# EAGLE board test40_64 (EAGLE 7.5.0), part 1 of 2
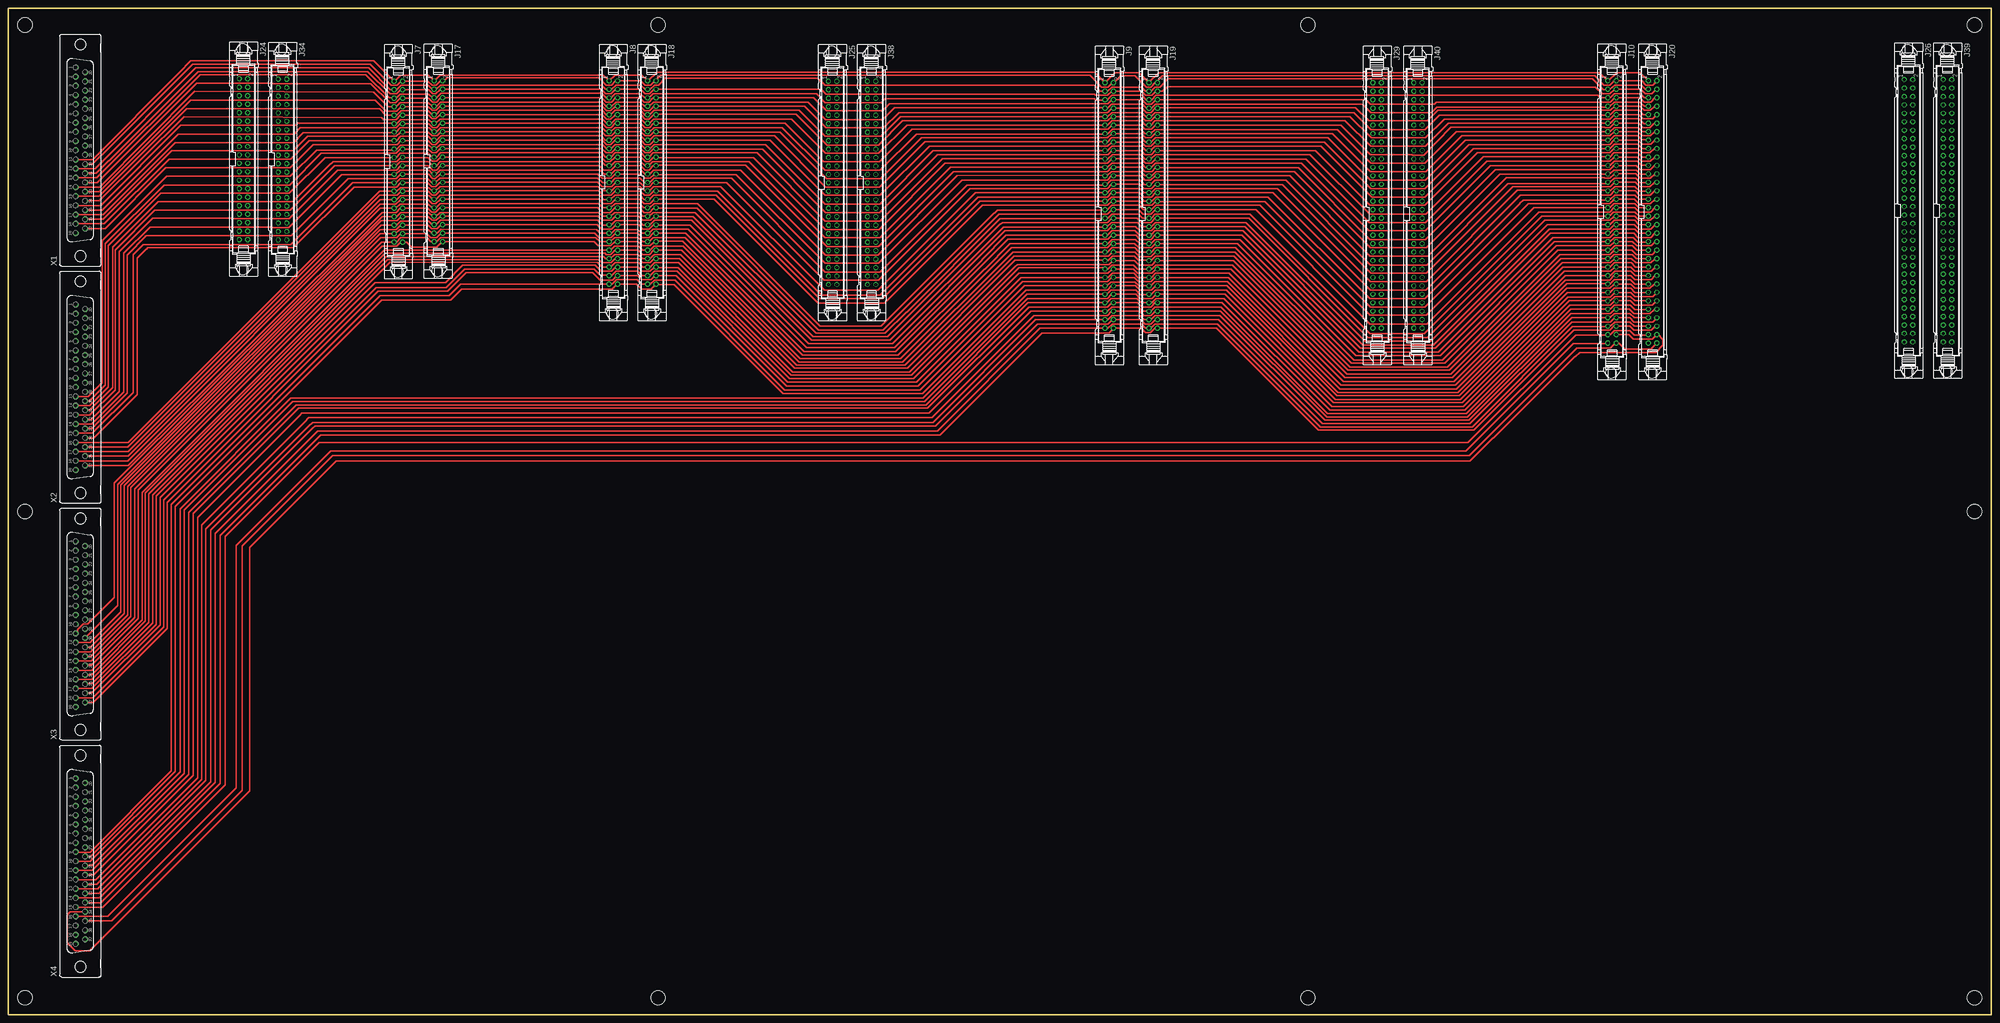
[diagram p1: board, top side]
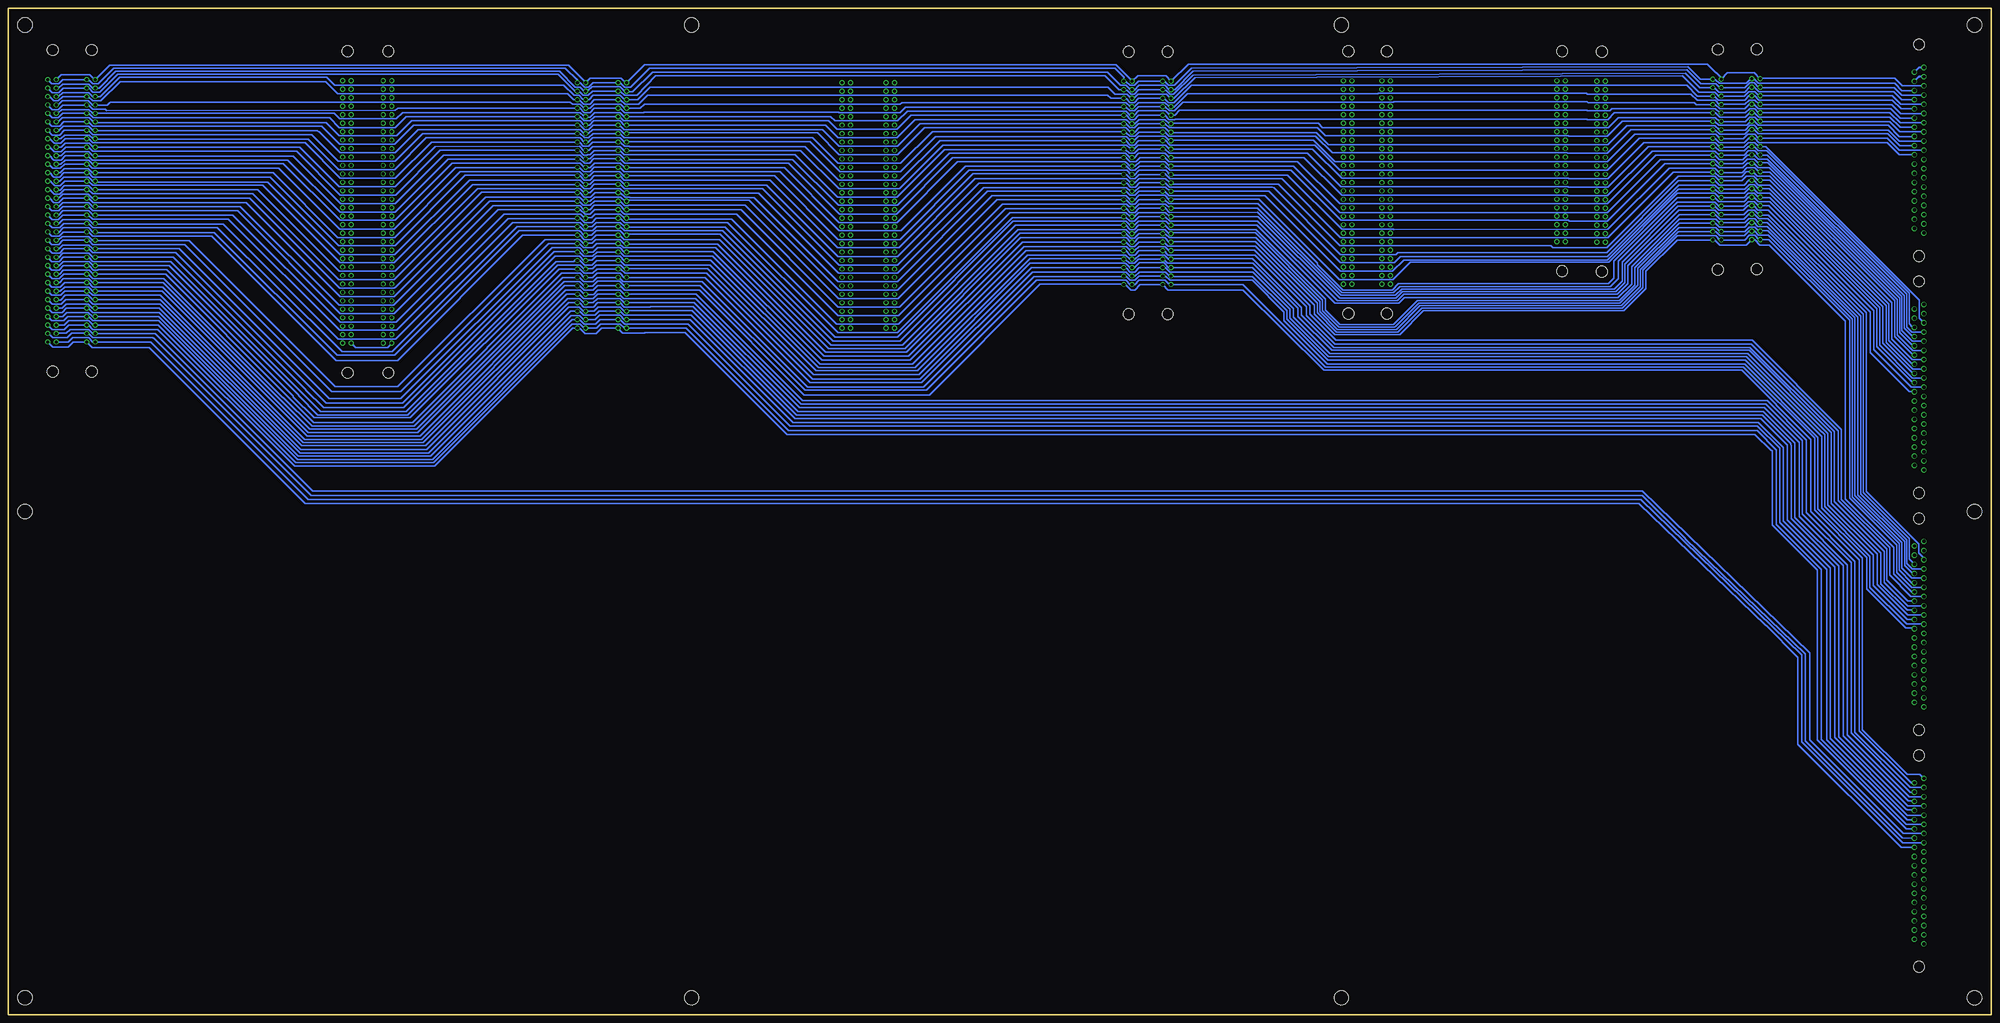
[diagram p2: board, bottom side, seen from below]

Size 595 x 302 mm. Coordinates in mm from the lower left corner, seen from the top.
Outline: 0,302 595,302 595,0 0,0 0,302
Copper layers (1*16): Top 0.035mm / dielectric 1.5mm / Bottom 0.035mm
Design rules "default": minimum track width 10mil, minimum drill 24mil, track to track 8mil, track to pad 8mil, pad to pad 8mil, via to via 8mil, smd to smd 8mil, copper to edge 40mil, drill to drill 8mil, minimum pad ring 10mil, minimum via ring 8mil, stop-mask expansion 4mil, vias tented up to drill 0mil, thermal gap 10mil
Holes 4.3 mm at 5,5 590,297 590,5 5,297 195,5 390,5 195,297 390,297 5,151 590,151

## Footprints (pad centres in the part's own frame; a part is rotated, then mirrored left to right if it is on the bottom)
40V = drill 0.914: 1 -24.13,-1.27 | drill 0.914 octagon: 2 -24.13,1.27; 3 -21.59,-1.27; 4 -21.59,1.27; 5 -19.05,-1.27; 6 -19.05,1.27; 7 -16.51,-1.27; 8 -16.51,1.27; 9 -13.97,-1.27; 10 -13.97,1.27; 11 -11.43,-1.27; 12 -11.43,1.27; 13 -8.89,-1.27; 14 -8.89,1.27; 15 -6.35,-1.27; 16 -6.35,1.27; 17 -3.81,-1.27; 18 -3.81,1.27; 19 -1.27,-1.27; 20 -1.27,1.27; 21 1.27,-1.27; 22 1.27,1.27; 23 3.81,-1.27; 24 3.81,1.27; 25 6.35,-1.27; 26 6.35,1.27; 27 8.89,-1.27; 28 8.89,1.27; 29 11.43,-1.27; 30 11.43,1.27; 31 13.97,-1.27; 32 13.97,1.27; 33 16.51,-1.27; 34 16.51,1.27; 35 19.05,-1.27; 36 19.05,1.27; 37 21.59,-1.27; 38 21.59,1.27; 39 24.13,-1.27; 40 24.13,1.27 | hole 3.302: 33.02,-0.254; -33.02,-0.254
50V = drill 0.914: 1 -30.48,-1.27 | drill 0.914 octagon: 2 -30.48,1.27; 3 -27.94,-1.27; 4 -27.94,1.27; 5 -25.4,-1.27; 6 -25.4,1.27; 7 -22.86,-1.27; 8 -22.86,1.27; 9 -20.32,-1.27; 10 -20.32,1.27; 11 -17.78,-1.27; 12 -17.78,1.27; 13 -15.24,-1.27; 14 -15.24,1.27; 15 -12.7,-1.27; 16 -12.7,1.27; 17 -10.16,-1.27; 18 -10.16,1.27; 19 -7.62,-1.27; 20 -7.62,1.27; 21 -5.08,-1.27; 22 -5.08,1.27; 23 -2.54,-1.27; 24 -2.54,1.27; 25 0,-1.27; 26 0,1.27; 27 2.54,-1.27; 28 2.54,1.27; 29 5.08,-1.27; 30 5.08,1.27; 31 7.62,-1.27; 32 7.62,1.27; 33 10.16,-1.27; 34 10.16,1.27; 35 12.7,-1.27; 36 12.7,1.27; 37 15.24,-1.27; 38 15.24,1.27; 39 17.78,-1.27; 40 17.78,1.27; 41 20.32,-1.27; 42 20.32,1.27; 43 22.86,-1.27; 44 22.86,1.27; 45 25.4,-1.27; 46 25.4,1.27; 47 27.94,-1.27; 48 27.94,1.27; 49 30.48,-1.27; 50 30.48,1.27 | hole 3.302: 39.37,-0.254; -39.37,-0.254
60V = drill 0.914: 1 -38.1,-1.27 | drill 0.914 octagon: 2 -38.1,1.27; 3 -35.56,-1.27; 4 -35.56,1.27; 5 -33.02,-1.27; 6 -33.02,1.27; 7 -30.48,-1.27; 8 -30.48,1.27; 9 -27.94,-1.27; 10 -27.94,1.27; 11 -25.4,-1.27; 12 -25.4,1.27; 13 -22.86,-1.27; 14 -22.86,1.27; 15 -20.32,-1.27; 16 -20.32,1.27; 17 -17.78,-1.27; 18 -17.78,1.27; 19 -15.24,-1.27; 20 -15.24,1.27; 21 -12.7,-1.27; 22 -12.7,1.27; 23 -10.16,-1.27; 24 -10.16,1.27; 25 -7.62,-1.27; 26 -7.62,1.27; 27 -5.08,-1.27; 28 -5.08,1.27; 29 -2.54,-1.27; 30 -2.54,1.27; 31 0,-1.27; 32 0,1.27; 33 2.54,-1.27; 34 2.54,1.27; 35 5.08,-1.27; 36 5.08,1.27; 37 7.62,-1.27; 38 7.62,1.27; 39 10.16,-1.27; 40 10.16,1.27; 41 12.7,-1.27; 42 12.7,1.27; 43 15.24,-1.27; 44 15.24,1.27; 45 17.78,-1.27; 46 17.78,1.27; 47 20.32,-1.27; 48 20.32,1.27; 49 22.86,-1.27; 50 22.86,1.27; 51 25.4,-1.27; 52 25.4,1.27; 53 27.94,-1.27; 54 27.94,1.27; 55 30.48,-1.27; 56 30.48,1.27; 57 33.02,-1.27; 58 33.02,1.27; 59 35.56,-1.27; 60 35.56,1.27
64V = drill 0.914: 1 -39.37,-1.27 | drill 0.914 octagon: 2 -39.37,1.27; 3 -36.83,-1.27; 4 -36.83,1.27; 5 -34.29,-1.27; 6 -34.29,1.27; 7 -31.75,-1.27; 8 -31.75,1.27; 9 -29.21,-1.27; 10 -29.21,1.27; 11 -26.67,-1.27; 12 -26.67,1.27; 13 -24.13,-1.27; 14 -24.13,1.27; 15 -21.59,-1.27; 16 -21.59,1.27; 17 -19.05,-1.27; 18 -19.05,1.27; 19 -16.51,-1.27; 20 -16.51,1.27; 21 -13.97,-1.27; 22 -13.97,1.27; 23 -11.43,-1.27; 24 -11.43,1.27; 25 -8.89,-1.27; 26 -8.89,1.27; 27 -6.35,-1.27; 28 -6.35,1.27; 29 -3.81,-1.27; 30 -3.81,1.27; 31 -1.27,-1.27; 32 -1.27,1.27; 33 1.27,-1.27; 34 1.27,1.27; 35 3.81,-1.27; 36 3.81,1.27; 37 6.35,-1.27; 38 6.35,1.27; 39 8.89,-1.27; 40 8.89,1.27; 41 11.43,-1.27; 42 11.43,1.27; 43 13.97,-1.27; 44 13.97,1.27; 45 16.51,-1.27; 46 16.51,1.27; 47 19.05,-1.27; 48 19.05,1.27; 49 21.59,-1.27; 50 21.59,1.27; 51 24.13,-1.27; 52 24.13,1.27; 53 26.67,-1.27; 54 26.67,1.27; 55 29.21,-1.27; 56 29.21,1.27; 57 31.75,-1.27; 58 31.75,1.27; 59 34.29,-1.27; 60 34.29,1.27; 61 36.83,-1.27; 62 36.83,1.27; 63 39.37,-1.27; 64 39.37,1.27 | hole 3.302: 48.26,-0.254; -48.26,-0.254
F37V = drill 1.016 octagon: 1 24.841,1.422; 2 22.073,1.422; 3 19.329,1.422; 4 16.561,1.422; 5 13.792,1.422; 6 11.049,1.422; 7 8.28,1.422; 8 5.512,1.422; 9 2.769,1.422; 10 0,1.422; 11 -2.769,1.422; 12 -5.512,1.422; 13 -8.28,1.422; 14 -11.049,1.422; 15 -13.818,1.422; 16 -16.561,1.422; 17 -19.329,1.422; 18 -22.098,1.422; 19 -24.841,1.422; 20 23.47,-1.422; 21 20.701,-1.422; 22 17.932,-1.422; 23 15.189,-1.422; 24 12.421,-1.422; 25 9.652,-1.422; 26 6.909,-1.422; 27 4.14,-1.422; 28 1.372,-1.422; 29 -1.372,-1.422; 30 -4.14,-1.422; 31 -6.909,-1.422; 32 -9.677,-1.422; 33 -12.421,-1.422; 34 -15.189,-1.422; 35 -17.958,-1.422; 36 -20.701,-1.422; 37 -23.47,-1.422 | hole 3.302: 31.75,0; -31.75,0

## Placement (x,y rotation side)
J7  [40V]  117.06,255.98 270 top
J8  [50V]  181.56,249.74 270 top
J9  60V  [60V]  330.38,241.56 270 top
J10  [64V]  481.2,240.88 270 top
J17  [40V]  129.03,256.11 270 top
J18  [50V]  193.13,249.74 270 top
J19  60V  [60V]  343.58,241.56 270 top
J20  [64V]  493.4,240.88 270 top
J24  [40V]  70.59,256.73 270 top
J25  [50V]  247.33,249.61 270 top
J26  [64V]  570.23,241.25 270 top
J29  60V  [60V]  410.78,241.56 270 top
J34  [40V]  82.31,256.63 270 top
J38  [50V]  259.03,249.61 270 top
J39  [64V]  581.93,241.25 270 top
J40  60V  [60V]  422.98,241.56 270 top
X1  [F37V]  21.63,259.4 90 top
X2  [F37V]  21.63,188.28 90 top
X3  [F37V]  21.63,117.16 90 top
X4  [F37V]  21.63,46.04 90 top

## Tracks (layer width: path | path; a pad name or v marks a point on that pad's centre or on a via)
1
  Bottom 0.406: X1.3 26.73,278.73 29,281 69.18,281 J24.1 69.36,280.86 71.12,282.62 79.17,282.62 J34.1 81.03,281.16 82.5,282.62 82.62,282.62 85.25,285.25 240.9,285.25 J25.1 246.06,280.19 247.62,281.75 256.1,281.75 J38.1 257.76,280.26 262.62,285.12 | J29.1 409.79,279.67 411.12,281 420.38,281 J40.1
  Bottom 0.506: J40.1 421.71,279.83 426.88,285 564.58,285 J26.1 569.12,280.62 570.62,282.12 579.15,282.12 J39.1
  Bottom 0.51: 262.62,285.12 404.05,285.12 J29.1
2
  Bottom 0.406: X1.22 26.83,277.33 29,279.5 69.88,279.5 71.23,280.86 J24.2 72.14,280.86 73.5,279.5 81.62,279.5 82.75,280.62 83.44,280.62 J34.2 87.27,280.76 91,284.49 240,284 245.12,278.88 246.88,278.88 248,280 248.51,280 J25.2 255.91,280.09 257.12,278.88 258.5,278.88 259.62,280 260.21,280 J38.2 | J29.2 419.58,279.67 420.88,278.38 422.12,278.38 423.38,279.62 424.21,279.62 J40.2
  Bottom 0.506: J40.2 424.25,280.38 427.88,284 563.38,284 568,279.38 569.75,279.38 570.62,280.25 571.13,280.25 J26.2 578.63,280.62 579.88,279.38 581.96,279.38 J39.2
  Bottom 0.51: J38.2 260.3,281.3 263,284 402.62,284 408.25,278.38 410.12,278.38 411.38,279.62 412.01,279.62 J29.2
3
  Bottom 0.406: X1.4 26.84,275.96 29.12,278.25 69.25,278.25 J24.3 69.82,278.32 71.12,279.62 72.38,279.62 73.88,278.12 80.94,278.12 J34.3 81.47,278.22 82.62,279.38 87.14,279.38 91.38,283.61 239.5,283.12 245,277.62 245.99,277.62 J25.3 246.68,277.55 248,278.88 255.75,278.88 257.12,277.5 257.71,277.5 J38.3 | J29.3 410.12,277.12 411.5,278.5 419.88,278.5 421.12,277.25 421.58,277.25 J40.3 | J26.3 569.71,278.08 570.88,279.25 578.75,279.25 580,278 580.58,278 J39.3
  Bottom 0.506: J26.3 567.79,278.08 562.75,283.12 429.62,283.12 424.88,278.38 423.5,278.38 422.25,277.12 J40.3
  Bottom 0.51: J38.3 258.3,277.55 259.62,278.88 261.25,278.88 265.25,282.88 401.75,282.88 407.62,277 409.38,277 J29.3
4
  Bottom 0.406: X1.23 26.84,274.59 29.25,277 69.75,277 71.12,278.38 71.81,278.38 J24.4 | J24.4 71.86,278.26 | J24.4 72.56,278.32 74,276.88 81.75,276.88 82.88,278 83.36,278 J34.4 87.48,278.22 91.75,282.49 239.5,282 245.38,276.25 246.38,276.25 247.62,277.38 248.43,277.38 J25.4 255.82,277.55 257.12,276.25 258.12,276.25 259.38,277.5 260.25,277.5 J38.4 | J29.4 419.75,277.12 421,275.88 422.5,275.88 423.62,277 424.12,277 J40.4 | J26.4 578.54,278.08 579.88,276.75 581.87,276.75 J39.4
  Bottom 0.506: J40.4 424.88,277.12 430,282.25 562.25,282.25 567.62,276.88 569.62,276.88 570.75,278 571.42,278 J26.4
  Bottom 0.51: J38.4 261.8,277.55 266,281.75 400.75,281.75 406.38,276 406.5,275.88 410.12,275.88 411.25,277 411.93,277 J29.4
5
  Bottom 0.406: X1.5 27.07,273.19 29.62,275.75 69.29,275.75 J24.5 69.78,275.78 71,277 72.75,277 74.12,275.62 80.98,275.62 J34.5 81.68,275.68 82.88,276.88 87.76,276.88 92.62,281.74 239,281.25 245.25,275 J25.5 246.26,275.01 247.5,276.25 256,276.25 257.12,275.12 257.64,275.12 J38.5 | J29.5 410.08,274.58 411.38,275.88 419.5,275.88 420.75,274.62 421.67,274.62 J40.5 | J26.5 569.66,275.54 570.88,276.75 578.75,276.75 579.88,275.62 580.58,275.62 J39.5
  Bottom 0.506: J26.5 567.46,275.54 561.62,281.38 499.5,281.38 497.12,279 428.38,279 425.25,275.88 423.75,275.88 422.62,274.75 421.88,274.75 J40.5
  Bottom 0.51: J38.5 258.13,275.01 259.38,276.25 262.88,276.25 265,278.38 402.38,278.38 406.12,274.62 409.47,274.62 J29.5
6
  Bottom 0.406: X1.24 26.95,271.82 29.62,274.5 69.75,274.5 71,275.75 71.83,275.75 J24.6 72.72,275.78 74,274.5 81.88,274.5 82.88,275.5 83.39,275.5 J34.6 88.18,275.68 91.38,278.88 121.25,278.88 121.38,279 240,279 245.25,273.75 246.88,273.75 247.88,274.75 248.34,274.75 J25.6 255.87,275.01 257.12,273.75 258.38,273.75 259.5,274.88 260.17,274.88 J38.6 | J29.6 419.17,274.58 420.5,273.25 422.38,273.25 423.62,274.5 424.17,274.5 J40.6 | J26.6 578.71,275.54 580,274.25 581.38,274.25 582.62,275.5 583.16,275.5 J39.6
  Bottom 0.506: J40.6 425.33,274.58 427.12,276.38 496.12,276.38 499.75,280 561.5,280 567.25,274.25 569.75,274.25 571,275.5 571.46,275.5 J26.6
  Bottom 0.51: J38.6 264.13,275.01 265.12,276 327.88,276 328,275.88 403.25,275.88 405.88,273.25 410,273.25 411.25,274.5 411.96,274.5 J29.6
7
  Bottom 0.406: X1.6 27.2,270.45 29.88,273.12 69.2,273.12 J24.7 69.61,273.24 70.88,274.5 72.62,274.5 73.88,273.25 80.92,273.25 J34.7 81.52,273.14 82.75,274.38 88.25,274.38 90.12,276.25 121.25,276.25 121.5,276.5 183.88,276.5 184,276.38 241.25,276.38 245.25,272.38 245.97,272.38 J25.7 246.59,272.47 247.88,273.75 255.88,273.75 257.25,272.38 257.67,272.38 J38.7 | J29.7 410.05,272.05 411.25,273.25 419.25,273.25 420.5,272 421.67,272 J40.7 | J26.7 569.75,273 571,274.25 578.88,274.25 579.88,273.25 580.41,273.25 J39.7
  Bottom 0.506: J26.7 565.38,273 564.62,273.75 564.5,273.75 564.38,273.88 426.38,273.88 425.75,273.25 423.5,273.25 422.38,272.12 421.79,272.12 J40.7
  Bottom 0.51: J38.7 258.35,272.47 259.62,273.75 326.88,273.75 327.38,273.25 404.12,273.25 405.38,272 409.46,272 J29.7
8
  Bottom 0.406: X1.25 27.3,269.05 30.12,271.88 69.87,271.88 71.23,273.24 J24.8 72.64,273.24 74,271.88 81.5,271.88 82.75,273.12 83.56,273.12 J34.8 88.52,273.14 89.12,273.75 121,273.75 121.25,274 179.25,274 179.38,273.88 242.5,273.88 245.12,271.25 246.62,271.25 247.88,272.5 248.57,272.5 J25.8 255.91,272.47 257.12,271.25 258.5,271.25 259.62,272.38 260.2,272.38 J38.8 | J29.8 419.2,272.05 420.5,270.75 422.25,270.75 423.62,272.12 424.17,272.12 J40.8 | J26.8 578.62,273 580,271.62 581.83,271.62 J39.8
  Bottom 0.506: J26.8 571.38,272.88 570.88,272.88 569.75,271.75 566,271.75 565.5,271.25 478.88,271.38 478.08,272.05 J40.8
  Bottom 0.51: J29.8 411.42,272.05 410.12,270.75 404.38,270.75 404.25,270.88 345.88,270.88 345.75,270.75 327.38,270.75 325.75,272.38 260.39,272.38 J38.8
9
  Bottom 0.406: X1.7 27.3,267.68 30.38,270.75 69.27,270.75 J24.9 69.83,270.7 71,271.88 72.5,271.88 73.75,270.62 81.01,270.62 J34.9 81.47,270.6 82.75,271.88 113.88,271.88 114.5,271.25 121.12,271.25 121.38,271.38 179.5,271.5 179.62,271.38 243.62,271.38 245,270 245.99,270 J25.9 246.43,269.93 247.75,271.25 255.88,271.25 257.12,270 257.69,270 J38.9 | J29.9 410.25,269.5 411.5,270.75 419.12,270.75 420.5,269.38 421.58,269.38 J40.9 | J26.9 569.71,270.46 570.88,271.62 579,271.62 580,270.62 580.5,270.62 J39.9
  Bottom 0.506: J40.9 421.95,269.75 422.38,269.75 423.38,270.75 476.75,270.75 478.62,268.88 495.62,268.88 | 495.75,268.88 495.62,268.88 | J26.9 497.21,270.46 495.62,268.88
  Bottom 0.51: J38.9 258.43,269.93 259.62,271.12 325.25,271.12 328.12,268.25 347,268.25 348.25,269.5 J29.9
10
  Bottom 0.406: X1.26 27.31,266.31 30.38,269.38 69.75,269.38 71.12,270.75 71.81,270.75 J24.10 72.42,270.7 73.75,269.38 81.5,269.38 82.75,270.62 83.55,270.62 J34.10 113.03,270.6 115,268.62 121.25,268.62 121.38,268.75 244.88,268.75 245,268.62 246.75,268.62 248,269.88 248.54,269.88 J25.10 255.82,269.93 257.12,268.62 258.25,268.62 259.5,269.88 260.25,269.88 J38.10 | J29.10 419.12,269.5 420.38,268.25 422.25,268.25 423.5,269.5 J40.10 | J26.10 578.66,270.46 580,269.12 581.87,269.12 J39.10
  Bottom 0.506: J40.10 475.62,269.5 478.88,266.25 495.75,266.25 498.62,269.12 569.5,269.12 570.88,270.5 571.46,270.5 J26.10
  Bottom 0.51: J29.10 411.63,269.5 410.38,268.25 348.88,268.25 346.38,265.75 328.38,265.75 324.12,270 260.37,270 J38.10
11
  Bottom 0.406: X1.8 27.41,264.91 30.5,268 69.16,268 J24.11 69.78,268.16 71,269.38 72.38,269.38 73.75,268 80.97,268 J34.11 81.56,268.06 82.75,269.25 111.88,269.25 114.88,266.25 200.62,266.25 201.88,267.5 245.95,267.5 J25.11 246.64,267.39 247.88,268.62 255.75,268.62 257.12,267.25 257.62,267.25 J38.11 | J29.11 410.21,266.96 411.5,268.25 419.38,268.25 420.62,267 421.68,267 J40.11 | J26.11 569.54,267.92 570.75,269.12 578.88,269.12 580.12,267.88 580.62,267.88 J39.11
  Bottom 0.506: J40.11 422.21,266.96 423.5,268.25 474,268.25 478.5,263.75 495.75,263.75 499.62,267.62 568.66,267.62 J26.11
  Bottom 0.51: J38.11 258.26,267.39 259.38,268.5 259.5,268.5 259.62,268.62 322.88,268.62 328.38,263.12 346,263.12 349.75,266.88 409.42,266.88 J29.11
12
  Bottom 0.406: X1.27 27.54,263.54 30.88,266.88 69.88,266.88 71.12,268.12 71.83,268.12 J24.12 72.09,268.16 73.38,266.88 81.75,266.88 82.88,268 83.52,268 J34.12 110.69,268.06 115.12,263.62 126.75,263.62 126.88,263.75 199.75,263.75 202.12,266.12 246.62,266.12 247.88,267.38 248.59,267.38 J25.12 255.86,267.39 257.12,266.12 258.38,266.12 259.62,267.38 260.29,267.38 J38.12 | J29.12 419.54,266.96 420.88,265.62 422.12,265.62 423.38,266.88 424.16,266.88 J40.12 | J26.12 578.33,267.92 579.62,266.62 581.9,266.62 J39.12
  Bottom 0.506: J40.12 473.41,266.96 479.12,261.25 495.62,261.25 501,266.62 569.62,266.62 570.88,267.88 571.46,267.88 J26.12
  Bottom 0.51: J29.12 411.59,266.96 410.25,265.62 350.75,265.62 345.75,260.62 328.25,260.62 321.5,267.38 260.31,267.38 J38.12
13
  Bottom 0.406: X1.9 27.54,262.17 30.88,265.5 69.2,265.5 J24.13 69.87,265.62 71.12,266.88 72.38,266.88 73.75,265.5 81.02,265.5 J34.13 81.64,265.52 82.88,266.75 109.38,266.75 115,261.12 198.88,261.12 202.5,264.75 245.96,264.75 J25.13 246.6,264.85 247.88,266.12 255.75,266.12 257,264.88 257.74,264.88 J38.13 | J29.13 410.3,264.43 411.5,265.62 419.75,265.62 420.88,264.5 421.63,264.5 J40.13 | J26.13 569.63,265.38 570.88,266.62 578.5,266.62 579.88,265.25 580.53,265.25 J39.13
  Bottom 0.506: J40.13 422.18,264.43 423.38,265.62 472,265.62 479,258.62 495.38,258.62 501.75,265 502,265 502.25,265.25 568.83,265.25 J26.13
  Bottom 0.51: J38.13 258.35,264.85 259.62,266.12 320.12,266.12 328.25,258.12 345.75,258.12 352.25,264.62 409.31,264.62 J29.13
14
  Bottom 0.406: X1.28 27.4,260.77 31,264.38 69.88,264.38 71.12,265.62 J24.14 72.63,265.62 74,264.25 81.5,264.25 82.75,265.5 83.56,265.5 J34.14 108.11,265.52 115.12,258.5 127.12,258.5 127.25,258.62 197.75,258.62 202.75,263.62 246.75,263.62 248,264.88 248.57,264.88 J25.14 255.78,264.85 257,263.62 258.5,263.62 259.62,264.75 260.2,264.75 J38.14 | J29.14 419.57,264.43 420.88,263.12 422.12,263.12 423.38,264.38 424.2,264.38 J40.14 | J26.14 578.25,265.38 579.62,264 581.82,264 J39.14
  Bottom 0.506: J40.14 470.7,264.43 479,256.12 496,256.12 504,264.12 569.62,264.12 570.88,265.25 571.37,265.25 J26.14
  Bottom 0.51: J29.14 411.43,264.43 410.25,263.25 353.75,263.25 346,255.5 327.25,255.5 317.75,265 260.45,265 J38.14
15
  Bottom 0.406: X1.10 27.52,259.4 31.12,263 69.24,263 J24.15 69.83,263.08 71,264.25 73,264.25 74.38,262.88 80.93,262.88 J34.15 81.36,262.98 82.62,264.25 107,264.25 115.25,256 196.88,256 203.38,262.5 245.87,262.5 J25.15 246.56,262.31 247.88,263.62 255.88,263.62 257.25,262.25 257.7,262.25 J38.15 | J29.15 410.13,261.88 411.38,263.12 419.75,263.12 421,261.88 J40.15 | J26.15 569.59,262.84 570.75,264 578.12,264 579.25,262.88 580.62,262.88 J39.15
  Bottom 0.506: J40.15 422.26,261.88 423.5,263.12 469.62,263.12 479.12,253.62 495.88,253.62 505,262.75 568.87,262.75 J26.15
  Bottom 0.51: J38.15 258.31,262.31 259.5,263.5 316.75,263.5 327.25,253 345.5,253 354.5,262 409.39,262 J29.15
16
  Bottom 0.406: X1.29 27.53,258.03 31.25,261.75 69.75,261.75 71,263 71.78,263 J24.16 72.8,263.08 74.12,261.75 81.62,261.75 82.75,262.88 83.47,262.88 J34.16 105.64,262.98 115.25,253.38 126.75,253.38 126.88,253.5 195.5,253.5 203,261 246.38,261 247.75,262.38 248.53,262.38 J25.16 255.81,262.31 257.12,261 258.38,261 259.62,262.25 260.24,262.25 J38.16 | J29.16 419.62,261.88 420.88,260.62 422.5,260.62 423.5,261.62 | 423.75,261.88 J40.16 | J26.16 577.91,262.84 579.25,261.5 581.25,261.5 582.62,262.88 583.16,262.88 J39.16
  Bottom 0.506: J26.16 570.84,262.84 569.62,261.62 506,261.62 495.38,251 478.88,251 468,261.88 423.75,261.88 423.5,261.62
  Bottom 0.51: J38.16 315.44,262.31 327.38,250.38 345.88,250.38 356,260.5 408.62,260.5 408.75,260.62 410.12,260.62 411.25,261.75 411.92,261.75 J29.16
17
  Bottom 0.406: X2.3 20.23,207.61 21.62,209 21.62,214.5 67.62,260.5 69.28,260.5 J24.17 69.79,260.54 71,261.75 72.88,261.75 74.25,260.38 80.97,260.38 J34.17 81.56,260.44 82.75,261.62 104.25,261.62 115,250.88 126.75,250.88 126.88,251 194.88,251 203.62,259.75 246.04,259.75 J25.17 246.52,259.77 247.75,261 256,261 257.12,259.88 257.65,259.88 J38.17 | J29.17 410.22,259.35 411.38,260.5 419.62,260.5 420.75,259.38 421.68,259.38 J40.17 | J26.17 569.55,260.3 570.75,261.5 578,261.5 579.12,260.38 580.59,260.38 J39.17
  Bottom 0.506: J40.17 422.35,259.35 423.62,260.62 466.88,260.5 478.88,248.5 495.75,248.5 507.62,260.38 568.88,260.38 J26.17
  Bottom 0.51: J29.17 357.22,259.35 345.75,247.88 327.62,247.88 314.5,261 259.5,261 258.5,260 257.99,260 J38.17
18
  Bottom 0.406: X2.22 23.21,206.38 23.62,206.38 24.62,207.38 24.62,216.5 67.38,259.25 69.88,259.25 71,260.38 71.69,260.38 J24.18 72.83,260.54 74.12,259.25 81.62,259.25 82.75,260.38 83.51,260.38 J34.18 102.94,260.44 115,248.38 126.88,248.38 127,248.5 195.12,248.5 205.12,258.5 246.62,258.5 247.88,259.75 248.58,259.75 J25.18 255.85,259.77 257.12,258.5 258.62,258.5 259.75,259.62 260.15,259.62 J38.18 | J29.18 419.28,259.35 420.5,258.12 421.25,258.12 421.38,258 422.38,258 423.62,259.25 424.15,259.25 J40.18 | J26.18 577.83,260.3 579.12,259 581.25,259 582.62,260.38 583.12,260.38 J39.18
  Bottom 0.506: J26.18 570.92,260.3 569.75,259.12 508.5,259.12 495.38,246 478.75,246 465.38,259.38 424.28,259.38 J40.18
  Bottom 0.51: J29.18 411.47,259.35 410.25,258.12 358.88,258.12 346.12,245.38 328.38,245.38 314.12,259.62 260.44,259.62 J38.18
19
  Bottom 0.406: X2.4 23.84,204.84 25.38,206.38 25.38,216.25 67.12,258 J24.19 69.75,258 71,259.25 72.88,259.25 74.12,258 80.94,258 J34.19 81.65,257.9 82.88,259.12 101.75,259.12 115.12,245.75 126.88,245.75 127,245.88 194.88,245.88 206.25,257.25 246.04,257.25 J25.19 246.6,257.23 247.88,258.5 255.88,258.5 257.12,257.25 257.74,257.25 J38.19 | J29.19 410.18,256.81 411.5,258.12 419.25,258.12 420.5,256.88 421.64,256.88 J40.19 | J26.19 569.63,257.76 570.88,259 577.88,259 579.12,257.75 J39.19
  Bottom 0.506: J40.19 422.31,256.81 423.5,258 464.38,258 479,243.38 495.25,243.38 509.5,257.62 568.83,257.62 J26.19
  Bottom 0.51: J38.19 258.48,257.23 259.75,258.5 312.62,258.5 328.25,242.88 345.88,242.88 359.62,256.62 409.33,256.62 J29.19
20
  Bottom 0.406: X2.23 23.59,203.47 26.12,206 26.12,215.75 67.12,256.75 69.88,256.75 71.12,258 J24.20 73.12,258 74.5,256.62 81.62,256.62 82.75,257.75 83.42,257.75 J34.20 100.6,257.9 115.12,243.38 195.5,243.38 208.12,256 246.75,256 248,257.25 248.58,257.25 J25.20 255.4,257.23 256.62,256 258.5,256 259.62,257.12 260.19,257.12 J38.20 | J29.20 419.32,256.81 420.62,255.5 422.12,255.5 423.38,256.75 423.75,256.75 424.19,256.75 J40.20 | J26.20 577.87,257.76 579.12,256.5 581.38,256.5 582.62,257.75 J39.20
  Bottom 0.506: J26.20 571.13,257.76 569.88,256.5 511.12,256.5 495.5,240.88 478.88,240.88 463,256.75 423.75,256.75
  Bottom 0.51: J29.20 411.43,256.81 410.12,255.5 360.88,255.5 345.62,240.25 328.5,240.25 311.62,257.12 260.4,257.12 J38.20
21
  Bottom 0.406: X2.5 23.7,202.07 26.88,205.25 26.88,215.5 67,255.62 69.16,255.62 J24.21 69.83,255.46 71.12,256.75 73.12,256.75 74.5,255.38 81.02,255.38 J34.21 81.73,255.36 83,256.62 99.25,256.62 115.25,240.62 126.88,240.62 127,240.75 195.5,240.75 209.38,254.62 246,254.62 J25.21 246.56,254.69 247.88,256 255.5,256 256.88,254.62 257.69,254.62 J38.21 | J29.21 410.14,254.26 411.38,255.5 419.12,255.5 420.5,254.12 421.57,254.12 J40.21 | 569.5,255.12 570.88,256.5 578,256.5 579.25,255.25 580.63,255.25 J39.21
  Bottom 0.506: J40.21 422.26,254.26 423.5,255.5 461.88,255.5 479,238.38 495.5,238.38 512.5,255.38 569.25,255.38 569.5,255.12 569.05,255.12 J26.21
  Bottom 0.51: J38.21 258.44,254.69 259.62,255.88 259.75,255.88 259.88,256 310.12,256 328.38,237.75 345.75,237.75 362.12,254.12 409.37,254.12 J29.21
22
  Bottom 0.406: X2.24 23.45,200.7 27.5,204.75 27.5,215 66.62,254.12 69.88,254.12 71.12,255.38 71.78,255.38 J24.22 73.17,255.46 74.5,254.12 81.62,254.12 82.75,255.25 83.47,255.25 J34.22 97.89,255.36 115.12,238.12 126.62,238.12 126.88,238.38 195.12,238.38 210.12,253.38 246.5,253.38 247.75,254.62 248.53,254.62 J25.22 255.56,254.69 256.88,253.38 258.25,253.38 259.5,254.62 260.24,254.62 J38.22 | J29.22 419.24,254.26 420.5,253 422.38,253 423.62,254.25 424.24,254.25 J40.22 | J39.22 582.85,255.22 581.62,254 579.38,254 578.12,255.25 571.53,255.25 J26.22
  Bottom 0.506: J26.22 571.1,255.22 569.88,254 513.88,254 495.62,235.75 479.25,235.75 460.75,254.25 424.26,254.25 J40.22
  Bottom 0.51: J29.22 411.51,254.26 410.25,253 363.5,253 345.75,235.25 327.12,235.25 307.75,254.62 260.37,254.62 J38.22
23
  Bottom 0.406: X2.6 23.58,199.33 28.25,204 28.25,214.62 66.5,252.88 69.28,252.88 J24.23 69.8,252.92 71,254.12 73.38,254.12 74.75,252.75 80.97,252.75 J34.23 81.69,252.82 82.88,254 96.62,254 115,235.75 179.25,235.62 179.38,235.75 194.88,235.75 211.12,252 245.91,252 J25.23 246.4,252.15 247.62,253.38 255.75,253.38 257.12,252 257.61,252 J38.23 | J29.23 410.35,251.72 411.62,253 419.38,253 420.62,251.75 421.69,251.75 J40.23 | J26.23 569.8,252.68 571,253.88 578.25,253.88 579.5,252.62 580.61,252.62 J39.23
  Bottom 0.506: J40.23 422.35,251.72 423.62,253 459.38,253 479.12,233.25 496.12,233.25 515.5,252.62 568.9,252.62 J26.23
  Bottom 0.51: J38.23 258.15,252.15 259.38,253.38 306.75,253.38 327.5,232.62 346,232.62 365.12,251.75 409.49,251.75 J29.23
24
  Bottom 0.406: X2.25 23.43,197.93 29,203.5 29,214.25 66.38,251.62 70.12,251.62 71.25,252.75 71.69,252.75 J24.24 73.45,252.92 74.88,251.5 81.62,251.5 82.88,252.75 83.5,252.75 J34.24 95.31,252.82 115,233.12 126.62,233.12 126.75,233.25 195.25,233.25 212.88,250.88 246.5,250.88 248,252.38 248.38,252.38 J25.24 255.72,252.15 257,250.88 258.25,250.88 259.5,252.12 260.27,252.12 J38.24 | J29.24 419.27,251.72 420.5,250.5 422.25,250.5 423.5,251.75 424.23,251.75 J40.24 | J26.24 578.32,252.68 579.62,251.38 581.38,251.38 582.62,252.62 583.14,252.62 J39.24
  Bottom 0.506: J26.24 570.93,252.68 569.62,251.38 516.5,251.38 495.88,230.75 479,230.75 457.88,251.88 424.4,251.88 J40.24
  Bottom 0.51: J29.24 411.48,251.72 410.25,250.5 366.5,250.5 346.12,230.12 327.75,230.12 305.5,252.38 260.52,252.38 J38.24
25
  Bottom 0.406: X2.7 23.68,196.56 29.88,202.75 29.88,213.75 66.5,250.38 J24.25 70,250.38 71.25,251.62 73.5,251.62 74.88,250.25 81,250.25 J34.25 81.53,250.28 82.88,251.62 93.88,251.62 115.38,230.12 131.5,230.12 132.12,230.75 195.38,230.75 213.88,249.25 245.7,249.25 J25.25 246.49,249.61 247.75,250.88 255.75,250.88 257,249.62 257.75,249.62 J38.25 | 328.25,227.5 346,227.5 346.62,228.12 | J29.25 410.19,249.19 411.5,250.5 419.25,250.5 420.5,249.25 421.64,249.25 J40.25 | J26.25 569.64,250.14 570.88,251.38 578.38,251.38 579.62,250.12 580.64,250.12 J39.25
  Bottom 0.506: J40.25 422.19,249.19 423.5,250.5 456.62,250.5 478.88,228.25 479,228.25 479.12,228.12 495.5,228.12 517.25,249.88 568.7,249.88 J26.25
  Bottom 0.51: J38.25 258.24,249.61 259.5,250.88 304.88,250.88 328.25,227.5 | 346.62,228.12 367.5,249 409.32,249 J29.25
26
  Bottom 0.406: X2.26 23.69,195.19 30.75,202.25 30.75,213.25 66.5,249 69.88,249 71.25,250.38 J24.26 72.75,250.38 74.12,249 81.62,249 82.88,250.25 83.55,250.25 J34.26 93.84,250.28 115.38,228.75 178,228.75 178.62,228.12 195.25,228.12 215.25,248.12 215.38,248.12 215.62,248.38 246.62,248.38 247.75,249.5 248.49,249.5 J25.26 255.51,249.61 256.75,248.38 258.25,248.38 259.38,249.5 260.19,249.5 J38.26 | J29.26 419.19,249.19 420.5,247.88 422.25,247.88 423.5,249.12 424.19,249.12 J40.26 | J26.26 578.11,250.14 579.5,248.75 581.12,248.75 582.5,250.12 583.18,250.12 J39.26
  Bottom 0.506: J26.26 571.01,250.14 569.75,248.88 518.62,248.88 495.38,225.62 479.25,225.62 455.75,249.12 424.31,249.12 J40.26
  Bottom 0.51: J29.26 411.44,249.19 410.12,247.88 368.62,247.88 345.75,225 328.12,225 318.75,234.38 318.75,234.5 303.75,249.5 260.41,249.5 J38.26
27
  Bottom 0.406: X2.8 23.54,193.79 31.5,201.75 31.5,212.75 66.62,247.88 69.28,247.88 J24.27 69.84,247.84 71.12,249.12 72.62,249.12 74,247.75 81.03,247.75 J34.27 81.61,247.74 82.88,249 93.75,249 115.25,227.5 177.25,227.5 179.12,225.62 195.25,225.62 216.75,247.12 246,247.12 J25.27 246.44,247.07 247.75,248.38 255.62,248.38 256.88,247.12 257.7,247.12 J38.27 258.32,247.07 259.5,248.25 302.38,248.25 328.25,222.5 345.88,222.5 369.88,246.5 409.37,246.5 J29.27 410.14,246.65 411.38,247.88 419.25,247.88 420.5,246.62 421.69,246.62 J40.27 | J26.27 569.73,247.6 570.88,248.75 578.25,248.75 579.5,247.5 580.56,247.5 J39.27
  Bottom 0.506: J40.27 422.27,246.65 423.5,247.88 454.25,247.88 479,223.12 495.75,223.12 520.25,247.62 568.93,247.62 J26.27
28
  Bottom 0.406: X2.27 23.42,192.42 32.5,201.5 32.5,212.5 66.5,246.5 70,246.5 71.25,247.75 71.77,247.75 J24.28 72.78,247.84 74.12,246.5 81.62,246.5 82.75,247.62 83.46,247.62 J34.28 93.89,247.74 115.12,226.5 176.25,226.5 179.62,223.12 195.25,223.12 217.88,245.75 246.75,245.75 248.07,247.07 J25.28 255.68,247.07 256.88,245.88 258.38,245.88 259.5,247 260.23,247 J38.28 301.18,247.07 328.25,220 346,220 371.25,245.25 408.5,245.25 408.62,245.38 410,245.38 411.38,246.75 411.94,246.75 J29.28 418.98,246.65 420.25,245.38 422.25,245.38 423.5,246.62 424.23,246.62 J40.28 | J26.28 578.27,247.6 579.62,246.25 581.25,246.25 582.5,247.5 583.1,247.5 J39.28
  Bottom 0.506: J26.28 570.98,247.6 569.75,246.38 521.62,246.38 495.88,220.62 479.25,220.62 453,246.88 424.48,246.88 J40.28
29
  Bottom 0.406: X2.9 23.67,191.05 33.5,200.88 33.5,212.25 66.5,245.25 69.27,245.25 J24.29 69.92,245.3 71.12,246.5 72.88,246.5 74.12,245.25 80.98,245.25 J34.29 81.58,245.2 82.88,246.5 94.12,246.5 114.75,225.88 174.25,225.88 179.5,220.62 195.62,220.62 219.75,244.75 245.84,244.75 J25.29 246.66,244.53 248,245.88 255.75,245.88 257.12,244.5 257.73,244.5 J38.29 258.4,244.53 259.62,245.75 299.88,245.75 328.25,217.38 345.75,217.38 372.75,244.38 409.24,244.38 J29.29 409.98,244.1 411.25,245.38 419.12,245.38 420.38,244.12 421.69,244.12 J40.29 | J26.29 569.81,245.06 571,246.25 578.62,246.25 579.75,245.12 580.6,245.12 J39.29
  Bottom 0.506: J40.29 422.36,244.1 423.5,245.25 423.62,245.25 423.75,245.38 451.75,245.38 479,218.12 479.12,218.12 479.25,218 495.62,218 522.62,245 568.9,245 J26.29
30
  Bottom 0.406: X2.28 23.53,189.65 34.38,200.5 34.38,211.88 66.5,244 69.88,244 71.12,245.25 71.81,245.25 J24.30 72.83,245.3 74.12,244 81.75,244 82.88,245.12 83.5,245.12 J34.30 94.17,245.2 113.25,226.12 113.25,221 114.88,219.38 177.88,219.38 179.75,217.5 194.5,217.5 202.12,225.12 202.12,225.5 220,243.38 246.75,243.38 247.88,244.5 248.57,244.5 J25.30 255.72,244.53 257,243.25 258.25,243.25 259.5,244.5 260.27,244.5 J38.30 | J29.30 419.14,244.1 420.38,242.88 422.5,242.88 423.62,244 424.14,244 J40.30 | J26.30 578.57,245.06 579.88,243.75 581.38,243.75 582.62,245 583.14,245 J39.30
  Bottom 0.506: J38.30 298.35,244.53 328,214.88 345.88,214.88 373.88,242.88 408.88,242.88 409,242.75 410.12,242.75 411.5,244.12 412.03,244.12 J29.30 | J26.30 570.93,245.06 569.75,243.88 569.62,243.88 569.5,243.75 523.62,243.75 495.38,215.5 479.25,215.5 450.62,244.12 424.27,244.12 J40.30
31
  Bottom 0.406: X2.10 23.91,188.28 35.25,199.62 35.25,211.25 66.75,242.75 J24.31 69.89,242.76 71.12,244 72.88,244 74.25,242.62 81,242.62 J34.31 81.78,242.66 83,243.88 94.12,243.88 111.88,226.12 111.88,220.88 114.25,218.5 177.5,218.5 179.38,216.62 194.88,216.62 194.88,216.75 220.12,242 J25.31 246.49,241.99 247.75,243.25 255.75,243.25 257,242 J38.31 | J29.31 410.19,241.56 411.5,242.88 419.25,242.88 420.5,241.62 421.65,241.62 J40.31 422.31,241.56 423.5,242.75 425.88,242.75 | J26.31 569.64,242.52 570.88,243.75 578.62,243.75 579.88,242.5 580.64,242.5 J39.31
  Bottom 0.506: J29.31 375.19,241.56 346,212.38 327.62,212.38 296.75,243.25 259.5,243.25 258.75,242.5 258.27,242.5 J38.31 | 425.88,242.75 449.5,242.75 479.38,212.88 495.75,212.88 525.38,242.5 568.94,242.5 J26.31
32
  Bottom 0.406: X2.29 24.53,186.91 36.25,198.62 36.25,210.88 66.88,241.5 70,241.5 71.12,242.62 71.72,242.62 J24.32 72.99,242.76 74.38,241.38 81.75,241.38 83,242.62 83.54,242.62 J34.32 93.97,242.66 110.75,225.88 110.75,220.12 113.12,217.75 176.88,217.75 178.75,215.88 195.12,215.88 220.12,240.88 246.62,240.75 247.88,242.12 248.47,242.12 J25.32 255.76,241.99 257,240.75 258.38,240.75 259.5,241.88 260.19,241.88 J38.32 | J29.32 419.06,241.56 420.38,240.25 422,240.25 423.38,241.62 424.19,241.62 J40.32 | J26.32 578.61,242.52 579.88,241.25 581.93,241.25 J39.32
  Bottom 0.506: J29.32 411.56,241.56 410.38,240.38 410.25,240.38 410.12,240.25 376.5,240.25 346,209.75 327.88,209.75 295.75,241.88 261.12,241.88 260.88,242.12 260.44,242.12 J38.32 | J26.32 570.89,242.52 569.62,241.25 526.25,241.25 495.38,210.38 479.25,210.38 448,241.62 424.31,241.62 J40.32
33
  Bottom 0.406: X3.3 20.21,136.96 21.75,138.5 21.75,141.25 37.5,157 37.5,210.62 66.88,240 69.1,240 J24.33 69.84,240.22 71.12,241.5 72.88,241.5 74.25,240.12 J34.33 81.62,240.12 82.88,241.38 93.75,241.38 109.88,225.25 109.88,219.75 112.62,217 176.62,217 178.62,215 195.5,215 220,239.5 246.01,239.5 J25.33 246.45,239.45 247.75,240.75 255.88,240.75 257.12,239.5 257.71,239.5 J38.33 | J29.33 410.15,239.03 411.38,240.25 418.88,240.25 420,239.12 421.61,239.12 J40.33 | 569,239.94 569.57,239.94 570.88,241.25 578.62,241.25 579.88,240 580.64,240 J39.33
  Bottom 0.506: J38.33 258.32,239.45 259.62,240.75 294.38,240.75 327.88,207.25 346.5,207.25 378,238.75 409.24,238.75 J29.33 | J40.33 422.02,239.03 423.25,240.25 446.25,240.25 478.62,207.88 495.5,207.88 527.62,240 568.5,240 569,239.5 569,239.94 J26.33
34
  Bottom 0.406: X3.22 23.05,135.18 24.62,136.75 24.62,142.88 38.38,156.62 38.38,210.25 67,238.88 69.75,238.88 71,240.12 71.77,240.12 J24.34 72.78,240.22 74.25,238.75 81.38,238.75 82.75,240.12 J34.34 93.63,240.12 109,224.75 109,219.38 112.12,216.25 176.25,216.25 178.25,214.25 196.25,214.25 220.12,238.12 246.5,238.12 247.75,239.38 248.53,239.38 J25.34 255.8,239.45 257.12,238.12 258.5,238.12 259.75,239.38 260.23,239.38 J38.34 | J29.34 418.6,239.03 419.88,237.75 422.12,237.75 423.38,239 424.23,239 J40.34 | J26.34 578.64,239.98 580,238.62 581.85,238.62 J39.34
  Bottom 0.506: J29.34 411.4,239.03 410.12,237.75 379.12,237.75 346,204.62 328.25,204.62 293.62,239.25 260.5,239.25 J38.34 | J26.34 570.98,239.98 569.75,238.75 529,238.75 495.62,205.38 478.5,205.38 445,238.88 424.4,238.88 J40.34
35
  Bottom 0.406: X3.4 23.72,133.72 25.38,135.38 25.38,142.5 39.12,156.25 39.12,209.62 67.25,237.75 69.25,237.75 J24.35 69.81,237.68 71,238.88 72.75,238.88 74,237.62 80.99,237.62 J34.35 81.45,237.58 82.62,238.75 93.62,238.75 107.88,224.5 107.88,219.25 112,215.12 176.12,215.12 177.75,213.5 197,213.5 220.38,236.88 246.03,236.88 J25.35 246.41,236.91 247.62,238.12 255.88,238.12 256.88,237.12 257.55,237.12 J38.35 | J29.35 410.11,236.49 411.38,237.75 418.62,237.75 419.88,236.5 421.69,236.5 J40.35 | J26.35 569.69,237.44 570.88,238.62 578.62,238.62 579.88,237.38 580.6,237.38 J39.35
  Bottom 0.506: J38.35 258.41,236.91 259.62,238.12 293.5,238.12 328.25,203.38 346.88,203.38 379.88,236.38 409.4,236.38 J29.35 | J40.35 422.24,236.49 423.5,237.75 443.75,237.75 478.75,202.75 496,202.75 530.5,237.25 568.77,237.25 J26.35
36
  Bottom 0.406: X3.23 23.6,132.35 26,134.75 26,142 40,156 40,209.38 67.12,236.5 70,236.5 71.12,237.62 71.81,237.62 J24.36 72.69,237.68 74,236.38 81.62,236.38 82.75,237.5 83.5,237.5 J34.36 93.55,237.58 106.88,224.25 106.88,219 111.62,214.25 172.25,214.25 179.38,207.12 195.38,207.12 199.75,211.5 199.75,214.75 220.62,235.62 246.62,235.62 247.88,236.88 248.56,236.88 J25.36 255.84,236.91 257.12,235.62 258.38,235.62 259.62,236.88 260.26,236.88 J38.36 | J29.36 418.51,236.49 419.75,235.25 422.25,235.25 423.5,236.5 424.24,236.5 J40.36 | 532.38,236.12 569.62,236.12 570.88,237.38 571.43,237.38 J26.36 578.31,237.44 579.62,236.12 581.88,236.12 J39.36
  Bottom 0.506: J29.36 411.36,236.49 410.12,235.25 380.62,235.25 347.5,202.12 327.5,202.12 292.75,236.88 260.33,236.88 J38.36 | J40.36 442.39,236.49 479.88,199 494.88,199 495.62,199.75 532.38,236.12
37
  Bottom 0.406: X3.5 23.83,130.95 26.88,134 26.88,141.75 40.88,155.75 40.88,209.12 67,235.25 69.21,235.25 J24.37 69.77,235.14 71,236.38 72.62,236.38 74,235 81,235 J34.37 81.42,235.04 82.62,236.25 93.75,236.25 106,224 106,218.88 111.38,213.5 171.75,213.5 178.75,206.5 178.88,206.5 179,206.38 195.75,206.38 200.62,211.25 200.62,214.5 220.75,234.62 245.81,234.62 J25.37 246.75,234.37 248,235.62 256,235.62 257.25,234.38 J38.37 | J29.37 410.07,233.94 411.38,235.25 418.62,235.25 420,233.88 421.64,233.88 J40.37 | J26.37 569.65,234.9 570.88,236.12 578.5,236.12 579.88,234.75 580.51,234.75 J39.37
  Bottom 0.506: J38.37 258.37,234.37 259.62,235.62 292,235.62 326.62,201 348.12,201 381.38,234.25 409.2,234.25 J29.37 | J40.37 422.32,233.94 423.5,235.12 423.62,235.12 423.75,235.25 441.75,235.25 479.12,197.88 496.38,197.88 533.25,234.75 568.81,234.75 J26.37
38
  Bottom 0.406: X3.24 23.83,129.58 27.62,133.38 27.62,141.38 41.62,155.38 41.62,208.75 66.88,234 69.88,234 71,235.12 71.84,235.12 J24.38 72.73,235.14 74.12,233.75 81.38,233.75 82.62,235 83.53,235 J34.38 93.83,235.04 105.25,223.62 105.25,218.5 111,212.75 171.38,212.75 178.5,205.62 196.12,205.62 201.5,211 201.5,214 220.62,233.12 246.62,233.12 247.75,234.25 248.48,234.25 J25.38 255.75,234.37 257.12,233 258.25,233 259.62,234.38 J38.38 | J29.38 418.68,233.94 420,232.62 422.25,232.62 423.5,233.88 424.18,233.88 J40.38 | J26.38 578.48,234.9 579.75,233.62 581.92,233.62 J39.38
  Bottom 0.506: J29.38 411.57,233.94 410.25,232.62 381.62,232.62 348.88,199.88 326,199.88 291.38,234.5 260.43,234.5 J38.38 | J26.38 570.9,234.9 569.62,233.62 534,233.62 496.62,196.25 478.25,196.25 440.62,233.88 424.32,233.88 J40.38
39
  Bottom 0.406: X3.6 23.83,128.21 28.38,132.75 28.38,140.88 42.5,155 42.5,208.38 66.75,232.62 69.3,232.62 J24.39 69.72,232.6 71,233.88 72.62,233.88 74,232.5 J34.39 81.38,232.5 82.62,233.75 94.12,233.75 104.5,223.38 104.5,218.25 110.75,212 170.88,212 178,204.88 196.5,204.88 202.25,210.62 202.25,213.5 220.75,232 245.89,232 J25.39 246.71,231.83 248,233.12 255.88,233.12 257.12,231.88 257.71,231.88 J38.39 | J29.39 410.28,231.41 411.5,232.62 418.75,232.62 419.88,231.5 421.62,231.5 J40.39 | 569,232.32 569.7,232.32 570.88,233.5 578.88,233.5 580,232.38 580.64,232.38 J39.39
  Bottom 0.506: J38.39 258.2,231.83 259.5,233.12 291.25,233.12 325.5,198.88 349.75,198.88 382.12,231.25 409.36,231.25 J29.39 | J40.39 422.4,231.41 423.62,232.62 434,232.62 478.12,188.5 497,188.5 540.75,232.25 568.85,232.25 J26.39 569,232.32
40
  Bottom 0.406: X3.25 23.81,126.81 29.25,132.25 29.25,140.25 43.75,154.75 43.75,208.12 66.62,231 69.38,231 71,232.62 71.83,232.62 J24.40 71.86,232.51 73.5,230.88 81.38,230.88 83,232.5 J34.40 94.25,232.5 103.62,223.12 103.62,217.88 110.25,211.25 170.38,211.25 177.5,204.12 197,204.12 203.12,210.25 203.12,213 220.75,230.62 247,230.62 248.12,231.75 248.52,231.75 J25.40 255.79,231.83 257.12,230.5 258.25,230.5 259.5,231.75 260.22,231.75 J38.40 | J29.40 418.47,231.41 419.75,230.12 422.38,230.12 423.5,231.25 424.1,231.25 J40.40 | 568.12,231.12 569.62,231.12 570.75,232.25 571.39,232.25 J26.40 578.64,232.36 579.88,231.12 581.97,231.12 J39.40
  Bottom 0.506: J29.40 411.65,231.41 410.38,230.12 382.75,230.12 350.25,197.62 324.88,197.62 290.62,231.88 260.35,231.88 J38.40 | 568.12,231.12 542.12,231.12 498,187 477.25,187 432.85,231.41 J40.40
41
  Bottom 0.406: X3.7 24.07,125.44 30.5,131.88 30.5,140.12 45,154.62 45,175.62 71.75,202.38 196.62,202.38 204.5,210.25 204.5,212.75 221.12,229.38 245.97,229.38 J25.41 246.79,229.29 248,230.5 255.75,230.5 256.88,229.38 257.68,229.38 J38.41 | J29.41 410.24,228.87 411.5,230.12 418.25,230.12 419.5,228.88 J40.41 | J26.41 569.7,229.82 570.88,231 578.62,231 579.75,229.88 580.61,229.88 J39.41
  Bottom 0.506: J38.41 258.29,229.29 259.5,230.5 290.25,230.5 324.38,196.38 350.88,196.38 383.5,229 409.38,229 J29.41 | J40.41 421.82,228.75 422.25,228.75 423.62,230.12 424.75,230.12 424.88,230.25 431.88,230.25 477.25,184.88 498.75,184.88 543.7,229.82 J26.41
42
  Bottom 0.406: X3.26 23.11,124.12 25,124.12 31.38,130.5 31.38,139.75 45.88,154.25 45.88,175.12 72,201.25 197,201.25 205.5,209.75 205.5,212.5 221,228 247,228 248.29,229.29 J25.42 255.71,229.29 257,228 258.38,228 259.5,229.12 260.13,229.12 J38.42 | J29.42 418.38,228.87 419.62,227.62 422.38,227.62 423.62,228.88 J40.42 | J26.42 578.3,229.82 579.62,228.5 581.88,228.5 J39.42
  Bottom 0.506: J29.42 411.49,228.87 410.25,227.62 383.75,227.62 351.38,195.25 323.62,195.25 289.62,229.25 259.62,229.25 259.5,229.12 | J26.42 570.95,229.82 569.75,228.62 544.75,228.62 499.62,183.5 476.75,183.5 431.25,229 424.38,229 J40.42
43
  Bottom 0.406: X3.8 25.05,122.67 32.12,129.75 32.12,139 47.12,154 47.12,175 72.38,200.25 197.25,200.25 207,210 207,212.25 221.62,226.88 245.94,226.88 J25.43 246.88,226.75 248.12,228 255.62,228 256.88,226.75 J38.43 | J29.43 410.2,226.32 411.5,227.62 418.62,227.62 419.88,226.38 421.66,226.38 J40.43 | J26.43 569.65,227.28 570.88,228.5 578.62,228.5 579.88,227.25 580.63,227.25 J39.43
  Bottom 0.506: J38.43 258.5,226.75 259.75,228 289.12,228 323,194.12 351.88,194.12 384.25,226.5 409.33,226.5 J29.43 | J40.43 422.32,226.32 423.62,227.62 430.88,227.62 476.38,182.12 500.38,182.12 505.75,187.5 505.75,187.62 545.5,227.38 568.87,227.38 J26.43
44
  Bottom 0.406: X3.27 23.13,121.38 25.25,121.38 33.12,129.25 33.12,138.5 48,153.38 48,174.75 72.62,199.38 197.88,199.38 208,209.5 208,212 221.5,225.5 247.12,225.5 248.38,226.75 J25.44 255.88,226.75 257.12,225.5 258.62,225.5 259.75,226.62 260.18,226.62 J38.44 | J29.44 418.55,226.32 419.88,225 422.12,225 423.38,226.25 424.18,226.25 J40.44 | J26.44 578.47,227.28 579.75,226 581.92,226 J39.44
  Bottom 0.506: J29.44 411.45,226.32 410.12,225 384.38,225 352.62,193.25 322.12,193.25 288.5,226.88 260.43,226.88 J38.44 | J26.44 570.9,227.28 569.62,226 546.25,226 501.25,181 475.62,181 430.62,226 425.38,226 425,226.38 424.3,226.38 J40.44
45
  Bottom 0.406: X3.9 25.05,119.93 34.25,129.12 34.25,138.25 49,153 49,174.38 73,198.38 198.38,198.38 209.38,209.38 209.38,211.88 221.62,224.12 245.97,224.12 J25.45 246.84,224.21 248.25,225.62 255.62,225.62 257.12,224.12 257.68,224.12 J38.45 | J29.45 410.04,223.78 411.25,225 418.62,225 419.75,223.88 421.62,223.88 J40.45 | J26.45 569.49,224.74 570.75,226 578.5,226 579.75,224.75 J39.45
  Bottom 0.506: J38.45 258.46,224.21 259.62,225.38 259.75,225.38 259.88,225.5 288.38,225.5 321.75,192.12 353.38,192.12 385.12,223.88 409.42,223.88 J29.45 | J40.45 422.16,223.78 423.38,225 430.12,225 475.12,180 502.12,180 507.88,185.75 507.88,185.88 546.75,224.75 J26.45
46
  Bottom 0.406: X3.28 23.15,118.62 25.25,118.62 35.38,128.75 35.38,137.88 50,152.5 50,174.12 50.75,174.88 50.88,174.88 73.5,197.5 198.88,197.5 210.38,209 210.38,211.75 221.5,222.88 246.5,222.88 247.84,224.21 J25.46 255.66,224.21 257,222.88 258.38,222.88 259.5,224 260.09,224 J38.46 | J29.46 418.34,223.78 419.62,222.5 422.25,222.5 423.5,223.75 424.21,223.75 J40.46 | J26.46 578.51,224.74 579.75,223.5 581.96,223.5 J39.46
  Bottom 0.506: J38.46 287.92,224.21 321.38,190.75 353.75,190.75 385.5,222.5 410,222.5 411.25,223.75 412.01,223.75 J29.46 | J26.46 571.38,224.62 570.62,224.62 569.5,223.5 568.12,223.5 568,223.62 547.5,223.62 509.5,185.62 509.5,185.38 503.25,179.12 474.38,179.12 429.71,223.78 J40.46
47
  Bottom 0.406: X3.10 25.29,117.16 36.38,128.25 36.38,137.5 50.88,152 50.88,173.5 73.75,196.38 199,196.38 211.38,208.75 211.38,211.25 221.62,221.5 245.89,221.5 J25.47 246.54,221.67 247.75,222.88 255.62,222.88 256.88,221.62 257.71,221.62 J38.47 | J29.47 410.25,221.25 411.5,222.5 418.38,222.5 419.62,221.25 J40.47 | J26.47 569.58,222.2 570.75,223.38 578.5,223.38 579.62,222.25 580.61,222.25 J39.47
  Bottom 0.506: J38.47 258.42,221.67 259.62,222.88 287.75,222.88 321,189.62 354.38,189.62 385.88,221.12 409.39,221.12 J29.47 | J40.47 422.25,221.25 423.5,222.5 429,222.5 473.75,177.75 503.38,177.75 511.12,185.5 | 511.12,185.5 511.12,185.38 | J26.47 547.83,222.2 511.12,185.5
48
  Bottom 0.406: X3.29 23.26,116 25.62,116 37.38,127.75 37.38,137.12 52,151.75 52,173.25 74,195.25 199.25,195.25 212.25,208.25 212.25,210.88 221.75,220.38 246.5,220.38 247.79,221.67 J25.48 255.71,221.67 257,220.38 258.38,220.38 259.5,221.5 260.13,221.5 J38.48 | J29.48 418.25,221.25 419.5,220 422.38,220 423.62,221.25 J40.48 | J26.48 578.42,222.2 579.75,220.88 581.88,220.88 J39.48
  Bottom 0.506: J29.48 411.75,221.25 410.5,220 386.88,220 355.25,188.38 320.38,188.38 287.25,221.5 260.47,221.5 J38.48 | J26.48 571.42,222.12 570.88,222.12 569.62,220.88 548.38,220.88 512.75,185.25 512.5,185.25 503.88,176.62 473.25,176.62 428.63,221.25 J40.48
49
  Bottom 0.406: X4.1 21.45,72.12 25.25,72.12 38.62,85.5 38.62,137 53,151.38 53,173 74.38,194.38 199.75,194.38 224.5,219.13 J25.49 246.63,219.13 247.88,220.38 255.75,220.38 257,219.12 J38.49 | J29.49 410.2,218.71 411.62,220.12 418.12,220.12 419.62,218.62 421.63,218.62 J40.49 | J26.49 569.66,219.66 570.88,220.88 578.5,220.88 579.62,219.75 580.57,219.75 J39.49
  Bottom 0.506: J38.49 258.38,219.13 259.62,220.38 286.5,220.38 319.5,187.38 356,187.38 387.38,218.75 409.46,218.75 J29.49 | J40.49 422.33,218.71 423.62,220 428.25,220 472.5,175.75 504.62,175.75 548.53,219.66 J26.49
50
  Bottom 0.406: X4.20 24.01,69.51 39.62,85.12 39.62,136.5 54.12,151 54.12,172.62 74.88,193.38 200.25,193.38 224.5,217.5 246.97,217.5 J25.50 255.37,219.13 257,217.5 258.12,217.5 259.62,219 260.17,219 J38.50 | J29.50 418.17,218.71 419.5,217.38 422.25,217.38 423.62,218.75 424.2,218.75 J40.50
  Bottom 0.506: J29.50 411.45,218.71 410.12,217.38 387.62,217.38 356.25,186 318.62,186 285.38,219.25 260.42,219.25 J38.50 | J40.50 428.05,218.71 472.12,174.62 505,174.62 548.75,218.38 569.62,218.38 570.91,219.66 J26.50 578.09,219.66 579.38,218.38 581.91,218.38 J39.50
51
  Bottom 0.406: X4.2 24.24,68.11 40.88,84.75 40.88,136 55.5,150.62 55.5,172.5 | 401.75,216.25 409.43,216.25 J29.51 410.17,216.16 411.38,217.38 418.12,217.38 419.38,216.12 421.67,216.12 J40.51
  Bottom 0.506: 401.75,216.25 388.62,216.25 356.62,184.25 67.25,184.25 55.5,172.5 | J40.51 422.29,216.16 423.5,217.38 427.75,217.38 471.5,173.62 505.38,173.62 548.87,217.12 J26.51 569.62,217.12 570.88,218.38 578.12,218.38 579.38,217.12 J39.51
52
  Bottom 0.406: J29.52 418.21,216.16 419.5,214.88 422.38,214.88 423.62,216.12 424.21,216.12 J40.52
  Bottom 0.506: 56.62,172.25 67.62,183.25 357.12,183.25 388.75,214.88 401.88,214.88 | J40.52 427.46,216.16 471,172.62 506.12,172.62 549.38,215.88 569.75,215.88 571,217.12 J26.52 578,217.12 579.25,215.88 581.96,215.88 J39.52
  Bottom 0.51: J29.52 411.67,216.16 410.38,214.88 401.88,214.88 | 56.62,172.25 56.62,150.25 42,135.62 42,84.5 24.25,66.75 X4.21
53
  Bottom 0.406: J29.53 410.25,213.62 411.5,214.88 418.25,214.88 419.5,213.62 J40.53
  Bottom 0.506: 402.38,213.75 389.25,213.75 357.62,182.12 68.12,182.12 57.62,171.62 | J40.53 422.38,213.62 423.62,214.88 427.25,214.88 470.5,171.62 506.5,171.62 549.46,214.58 J26.53 569.71,214.58 571,215.88 577.88,215.88 579.25,214.5 580.58,214.5 J39.53
  Bottom 0.51: X4.3 24.62,65.37 43.12,83.88 43.12,135 57.62,149.5 57.62,171.62 | 402.38,213.75 409.38,213.75 J29.53
54
  Bottom 0.506: 58.88,171.38 58.88,171.5 68.38,181 358,181 389.5,212.5 402.25,212.5 402.38,212.38 | J29.54 418.12,213.62 419.38,212.38 422.38,212.38 423.5,213.5 424.12,213.5 J40.54 426.88,213.62 469.75,170.75 507,170.75 549.5,213.25 569.75,213.25 571.08,214.58 J26.54 577.79,214.58 579.12,213.25 581.87,213.25 J39.54
  Bottom 0.51: J29.54 411.5,213.62 410.25,212.38 402.38,212.38 | 58.88,171.38 58.88,149.25 44.38,134.75 44.38,83.62 24.88,64.12 23.2,64.12 X4.22
55
  Bottom 0.406: J26.55 569.79,212.04 571,213.25 572.12,213.25
  Bottom 0.506: 402.75,211.25 389.88,211.25 358.5,179.88 68.62,179.88 60.12,171.38 60.12,171 60,170.88 | J29.55 410.21,211.09 411.5,212.38 418,212.38 419.25,211.12 421.67,211.12 J40.55 422.46,211.09 423.75,212.38 426.88,212.38 469.5,169.62 507.25,169.62 549.66,212.04 J26.55 | 572.12,213.25 577.62,213.25 578.88,212 580.62,212 J39.55
  Bottom 0.51: X4.4 24.98,62.6 45.75,83.38 45.75,134.62 60,148.88 60,170.88 | 402.75,211.25 409.35,211.25 J29.55
56
  Bottom 0.506: 61.12,170.5 61.12,170.88 69.12,178.88 359,178.88 390.12,210 403,210 403.12,209.88 | J29.56 417.79,211.09 419,209.88 422.38,209.88 423.5,211 424.17,211 J40.56 426.29,211.09 468.88,168.5 507.5,168.5 549.75,210.75 569.75,210.75 571.04,212.04 J26.56 571.54,212 577.62,212 578.88,210.75 581.88,210.75 583.16,212.04 J39.56
  Bottom 0.51: J29.56 411.46,211.09 410.25,209.88 403.12,209.88 | 61.12,170.5 61.12,148.5 47,134.38 47,83.12 25.5,61.62 25.38,61.62 25.25,61.5 23.32,61.5 X4.23
57
  Bottom 0.406: J26.57 569.75,209.5 571,210.75 577.5,210.75 578.75,209.5 J39.57
  Bottom 0.506: 403.5,208.62 390.38,208.62 359.5,177.75 69.88,177.75 62.38,170.25 | J29.57 410.17,208.54 411.5,209.88 417.62,209.88 418.88,208.62 421.63,208.62 J40.57 422.42,208.54 423.62,209.75 426.12,209.75 468.25,167.62 508,167.62 549.88,209.5 J26.57
  Bottom 0.51: X4.5 25.21,59.83 48.25,82.88 48.25,134 62.38,148.12 62.38,170.25 | 403.5,208.62 409.43,208.62 J29.57
58
  Bottom 0.506: 63.5,170 70.12,176.62 360.38,176.62 391,207.25 404.12,207.25 | J29.58 417.45,208.54 418.75,207.25 422.25,207.25 423.5,208.5 424.2,208.5 J40.58 425.83,208.54 467.75,166.62 508.25,166.62 549.88,208.25 569.62,208.25 570.88,209.5 J26.58 577.12,209.5 578.38,208.25 581.95,208.25 J39.58
  Bottom 0.51: J29.58 411.42,208.54 410.12,207.25 404.12,207.25 403.62,207.25 | 63.5,170 63.5,147.75 49.38,133.62 49.38,82.5 25.25,58.38 23.14,58.38 X4.24
59
  Bottom 0.506: 403.88,206 391.62,206 360.88,175.25 70.25,175.25 64.5,169.5 | J29.59 410.13,206 411.38,207.25 417.25,207.25 418.5,206 J40.59 422.25,206 423.5,207.25 425.88,207.25 467.38,165.75 508.75,165.75 549.96,206.96 J26.59 569.59,206.96 570.88,208.25 576.88,208.25 578.25,206.88 580.58,206.88 J39.59
  Bottom 0.51: X4.6 25.46,57.09 51,82.62 51,133.62 64.5,147.12 64.5,169.5 | 403.88,206 J29.59
60
  Bottom 0.506: 65.75,169.25 66,169.25 70.88,174.12 361.38,174.12 392,204.75 403.88,204.75 404.12,204.5 | J29.60 417,206 418.62,204.38 422,204.38 423.5,205.88 424.12,205.88 J40.60 425.75,206 467.12,164.62 509.12,164.62 550.12,205.62 569.62,205.62 570.88,206.88 J26.60 576.91,206.96 578.25,205.62 581.87,205.62 J39.60
  Bottom 0.51: J29.60 412.05,205.93 410.62,204.5 404.12,204.5 | 65.75,169.25 65.75,147 52.25,133.5 52.25,82.5 25.5,55.75 23.11,55.75 X4.25
61
  Bottom 0.506: X4.7 26.45,54.32 54.5,82.38 54.5,108.5 104.62,157.12 503.62,157.12 550.88,204.38 568.91,204.38 J26.61 569.67,204.42 570.88,205.62 576.5,205.62 577.62,204.5 580.58,204.5 J39.61
62
  Bottom 0.506: X4.26 26.62,53 55.75,82.12 55.75,108.25 91.75,142.75 91.75,142.88 104.62,155.75 504.12,155.75 551.38,203 551.5,203 551.62,203.12 569.62,203.12 571,204.5 571.42,204.5 J26.62 571.58,204.5 576,204.5 577.38,203.12 581.62,203.12 582.92,204.42 J39.62
63
  Bottom 0.506: X4.8 26.55,51.55 56.88,81.88 56.88,107.88 105.12,154.62 505,154.62 552.25,201.88 J26.63 | J26.63 | J26.63 569.63,201.88 570.88,203.12 575.75,203.12 577,201.88 J39.63
64
  Bottom 0.506: X4.27 23.11,50.12 27,50.12 58,81.12 58,107.25 67.5,116.75 67.62,116.75 105.75,153.38 505.88,153.38 552.75,200.25 569.87,200.25 J26.64 575.5,201.88 577,200.38 581.7,200.38 J39.64
+5V
  Bottom 0.61: X1.2 21.68,281.47 X1.21
GND
  Bottom 0.61: X1.1 21.68,284.24 X1.20
L1
  Top 0.406: X1.11 25.26,256.63 51.25,282.62 51.25,282.75 54.75,286.25 109.64,286.25 J7.1 115.86,280.11 117.75,282 125.99,282 J17.1 127.86,280.24 129.62,282 178.5,282 J8.1 180.28,280.29 182,282 190.07,282 J18.1 | J19.1 342.31,279.81 345.25,282.75
  Top 0.506: J9.1 329.11,279.74 332.12,282.75 339.23,282.75 J19.1 | 345.25,282.75 477.43,282.75 J10.1 480.12,280.25 482.62,282.75 489.63,282.75 J20.1
  Top 0.51: J18.1 191.97,280.21 194.62,282.88 325.9,282.88 J9.1
L2
  Top 0.406: X1.30 25.14,255.26 28,258.12 28.12,258.12 55.25,285.25 108.5,285.25 114.88,278.88 116.62,278.88 117.75,280 118.22,280 J7.2 125.89,280.11 127.12,278.88 128.38,278.88 129.62,280.12 130.19,280.12 J17.2 130.74,280.24 131.62,281.12 177.25,281.12 179.38,279 181,279 182.12,280.12 182.74,280.12 J8.2 189.78,280.21 191,279 192.75,279 193.88,280.12 194.31,280.12 J18.2
  Top 0.506: J9.2 331.79,279.67 333.88,281.75 338.12,281.75 341.5,278.38 342.88,278.38 344.12,279.62 344.81,279.62 J19.2 344.85,280.23 346.38,281.75 476,281.75 478.75,279 480.62,279 481.75,280.12 482.36,280.12 J10.2 490.13,280.25 491.38,279 493.43,279 J20.2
